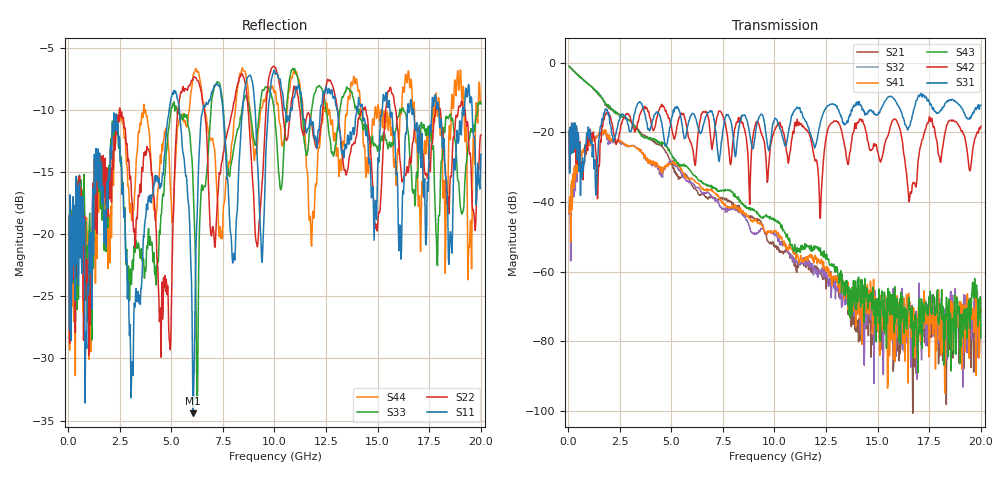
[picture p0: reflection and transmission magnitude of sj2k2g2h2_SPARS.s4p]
! FILE: E:\users\goganessyan\GBX_Backplane\FR408_backplane\1m_INBOUND_TRU\sj2k2g2h2_SPARS.s4p
# MHZ S RI R 50.00
! FREQ  S11  S12  S13  S14
!  S21  S22  S23  S24
!  S31  S32  S33  S34
!  S41  S42  S43  S44
!  REAL  IMAG  REAL  IMAG  REAL  IMAG  REAL  IMAG
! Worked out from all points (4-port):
!   799 points, 50 MHz to 20 GHz, reference 50 ohm
!   strongest paths, dB at 50 MHz, 5.025 GHz, 10.03 GHz, 15.03 GHz, 20 GHz:
!     S31: -19.7, -15.6, -15.9, -14.7, -12.2
!     S42: -19.7, -19.1, -19.3, -26.0, -18.3
!     S43: -1.1, -26.5, -45.5, -67.6, -79.0
!     S41: -42.8, -28.9, -48.5, -68.7, -71.3
!     S32: -43.5, -28.4, -49.0, -74.5, -78.9
!     S21: -1.0, -29.3, -53.0, -73.8, -71.6
!   lowest |S11| = -34.4 dB at 6.05 GHz (marker M1), VSWR 1.04, Z = 51.6 + j1.02 ohm
!   |S11| at or under -10 dB: start of sweep to 4.897 GHz; 5.39 GHz to 6.531 GHz (1.141 GHz wide, 19.1 % of centre); 17.96 GHz to 19.11 GHz (1.15 GHz wide, 6.2 % of centre)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
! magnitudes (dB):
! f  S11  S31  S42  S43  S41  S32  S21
! 50 MHz  -18.6  -19.7  -19.7  -1.1  -42.8  -43.5  -1.0
! 1.7 GHz  -16.1  -15.7  -17.1  -10.5  -20.1  -20.8  -10.6
! 6.05 GHz  -34.4  -14.6  -25.1  -32.1  -33.5  -34.7  -35.7
! 7.15 GHz  -8.0  -19.6  -17.8  -36.2  -38.0  -39.4  -39.1
! 12.22 GHz  -10.0  -17.1  -44.7  -53.2  -57.7  -60.3  -60.3
! 12.9 GHz  -8.9  -12.0  -16.7  -59.1  -61.3  -64.9  -61.6
! 20 GHz  -13.6  -12.2  -18.3  -79.0  -71.3  -78.9  -71.6
